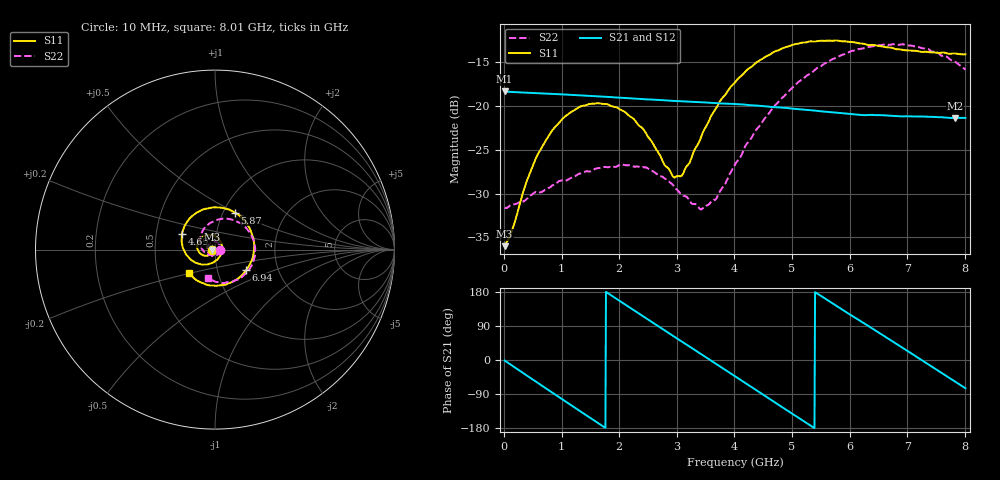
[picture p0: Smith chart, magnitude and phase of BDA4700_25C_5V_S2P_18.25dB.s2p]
!Agilent Technologies,E5071B,MY42404982,A.09.10
!Date: Mon Oct 20 13:35:27 2025
!Data & Calibration Information:
!Freq	S11:SOLT2(ON)	S21:SOLT2(ON)	S12:SOLT2(ON)	S22:SOLT2(ON)
# Hz S RI R 50
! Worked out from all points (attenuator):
!   801 points, 10 MHz to 8.01 GHz, reference 50 ohm
!   highest |S21| = -18.34 dB at 10 MHz (marker M1); lowest = -21.4 dB at 7.83 GHz (marker M2)
!   lowest |S11| = -36.0 dB at 10 MHz (marker M3), VSWR 1.03, Z = 48.4 - j0.122 ohm
!   |S11| at or under -10 dB: start of sweep to end of sweep
!   |S22| runs from -31.8 to -13.0 dB; largest |S21 - S12| = 0.00098
!   S11 on the Smith chart (normalised r, x): 10 MHz: 0.97, -0.00; 4.69 GHz: 0.68, +0.12; 5.87 GHz: 1.13, +0.49; 6.94 GHz: 1.38, -0.33; 8.01 GHz: 0.72, -0.20
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1e7  -0.0158 -0.00126  0.1211 -0.00261  0.121 -0.00271  0.0261 -0.000871
1.3e8  -0.0169 -0.00911  0.1168 -0.0285  0.1167 -0.0286  0.0265 -0.00635
3.8e8  -0.0261 -0.0249  0.0921 -0.0756  0.092 -0.0757  0.0212 -0.0199
6e8  -0.0419 -0.0339  0.0558 -0.1042  0.0557 -0.1043  0.0124 -0.0296
1e9  -0.0798 -0.0239  -0.0251 -0.1136  -0.0252 -0.1138  -0.0159 -0.0341
1.35e9  -0.0994 0.0105  -0.0852 -0.0769  -0.0852 -0.0769  -0.0378 -0.0168
2.07e9  -0.0461 0.0813  -0.0959 0.0562  -0.096 0.0562  -0.0286 0.0362
2.68e9  0.0304 0.0447  0.002 0.1082  0.00198 0.1082  0.0171 0.0364
2.94e9  0.0391 0.00448  0.0483 0.0953  0.0483 0.0952  0.0283 0.0208
3.08e9  0.0352 -0.0185  0.0694 0.0805  0.069 0.0807  0.0301 0.00908
3.45e9  -0.00652 -0.07  0.1023 0.023  0.1024 0.0229  0.0173 -0.0196
3.69e9  -0.052 -0.0831  0.1017 -0.0199  0.1018 -0.0202  -0.00233 -0.0295
4.01e9  -0.1192 -0.0661  0.0751 -0.0698  0.0751 -0.0697  -0.0368 -0.0278
4.69e9  -0.1844 0.0868  -0.0347 -0.0921  -0.0345 -0.0922  -0.0841 0.053
5.35e9  -0.0563 0.2264  -0.0941 -0.00672  -0.0941 -0.00698  -0.0135 0.1547
5.87e9  0.1095 0.2063  -0.0623 0.0662  -0.0623 0.0662  0.1083 0.1629
6.26e9  0.197 0.1101  -0.00926 0.0881  -0.00845 0.0881  0.1895 0.0997
6.68e9  0.213 -0.0337  0.0504 0.0721  0.0506 0.0722  0.2234 -0.00919
6.94e9  0.1744 -0.1139  0.0753 0.0437  0.0755 0.0434  0.2091 -0.0804
7.37e9  0.052 -0.1962  0.0848 -0.0177  0.0848 -0.018  0.1283 -0.1676
7.83e9  -0.1001 -0.172  0.0468 -0.0712  0.0468 -0.0714  0.00277 -0.1789
8.01e9  -0.1454 -0.1331  0.0228 -0.0823  0.0229 -0.0824  -0.0395 -0.1561
